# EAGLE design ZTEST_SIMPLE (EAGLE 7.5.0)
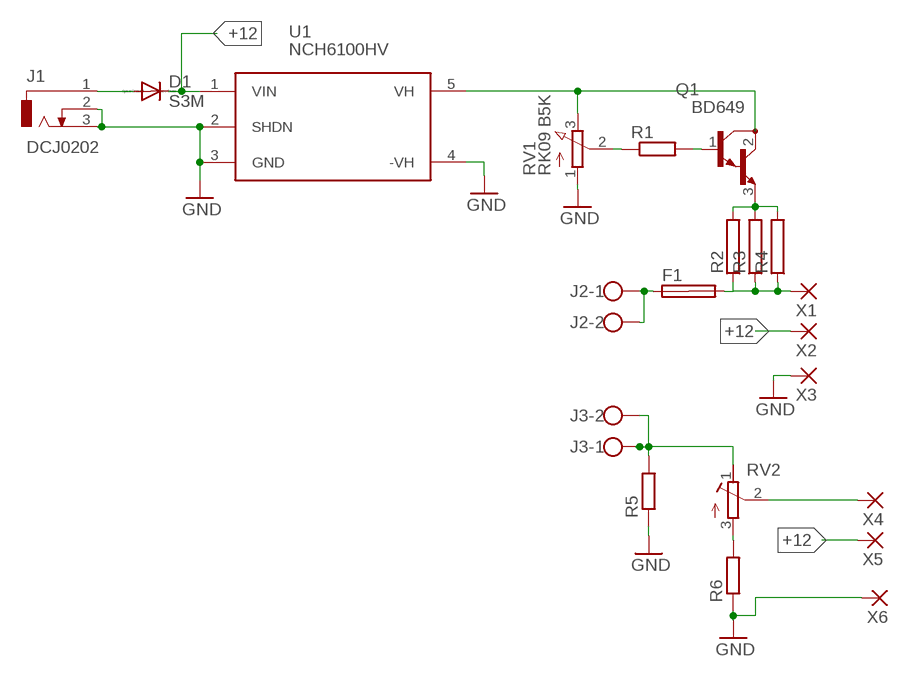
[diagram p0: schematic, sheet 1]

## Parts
D1  S3M  [SMC]
F1  SHK20L  [SHK20L]
J1  DCJ0202  [DCJ0202]
J2  W237-102  [W237-102]
J3  W237-102  [W237-102]
Q1  BD649  [TO220]
R1  R-EU_0207/10  [0207/10]
R2  RAC05  [AC05]
R3  RAC05  [AC05]
R4  RAC05  [AC05]
R5  R-EU_0411/12  [0411/12]
R6  R-EU_0207/10  [0207/10]
RV1  RK09 B5K  PV09A  [PTV09]
RV2  R-TRIMM-3386-F  [R-TRIMM-3386F]
U1  NCH6100HV  [NCH6100HV]
X1  2,54/1,1  [2,54/1,1]
X2  2,54/1,1  [2,54/1,1]
X3  2,54/1,1  [2,54/1,1]
X4  2,54/1,1  [2,54/1,1]
X5  2,54/1,1  [2,54/1,1]
X6  2,54/1,1  [2,54/1,1]

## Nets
+12: D1.C U1.1(VIN) X2.1(P) X5.1(P)
GND: J1.2 J1.3 R5.1 R6.1 RV1.1(A) U1.2(SHDN) U1.3(GND) U1.4(-VH) X3.1(P) X6.1(P)
N$2: D1.A J1.1
N$3: Q1.2(C) RV1.3(E) U1.5(VH)
N$4: Q1.1(B) R1.2
N$5: R1.1 RV1.2(S)
N$6: Q1.3(E) R2.2 R3.2 R4.2
N$7: F1.2A R2.1 R3.1 R4.1 X1.1(P)
N$8: F1.1A J2.1 J2.2
N$9: J3.1 J3.2 R5.2 RV2.1(A)
N$32: R6.2 RV2.3(E)
N$33: RV2.2(S) X4.1(P)
Unconnected: F1.1B F1.2B

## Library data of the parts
D1 = diode:S3M
F1 = fuse:SHK20L: FUSE HOLDER 5 x 20 mm, SH contact, SHH1 Schukat, E1073 Buerklin; OC_FARNELL: unknown; OC_NEWARK: unknown
J1 = con-jack:DCJ0202: DC POWER JACK Source: DCJ0202.pdf; OC_FARNELL: unknown; OC_NEWARK: unknown
J2 J3 = con-wago-500:W237-102: WAGO SCREW CLAMP; MPN: 237-102; OC_FARNELL: unknown; OC_NEWARK: 70K9898
Q1 = transistor:BD649: NPN BIPOLAR DARLINGTON TRANSISTOR
R1 R5 R6 = rcl:R-EU_: RESISTOR, European symbol
R2-R4 = resistor-power:R: Power Resitor; OC_FARNELL: unknown; OC_NEWARK: unknown
RV1 = pot:PV09A
RV2 = rcl:R-TRIMM-3386-F
U1 = dc-dc-converter:NCH6100HV
X1-X6 = wirepad:2,54/1,1: THROUGH-HOLE PAD

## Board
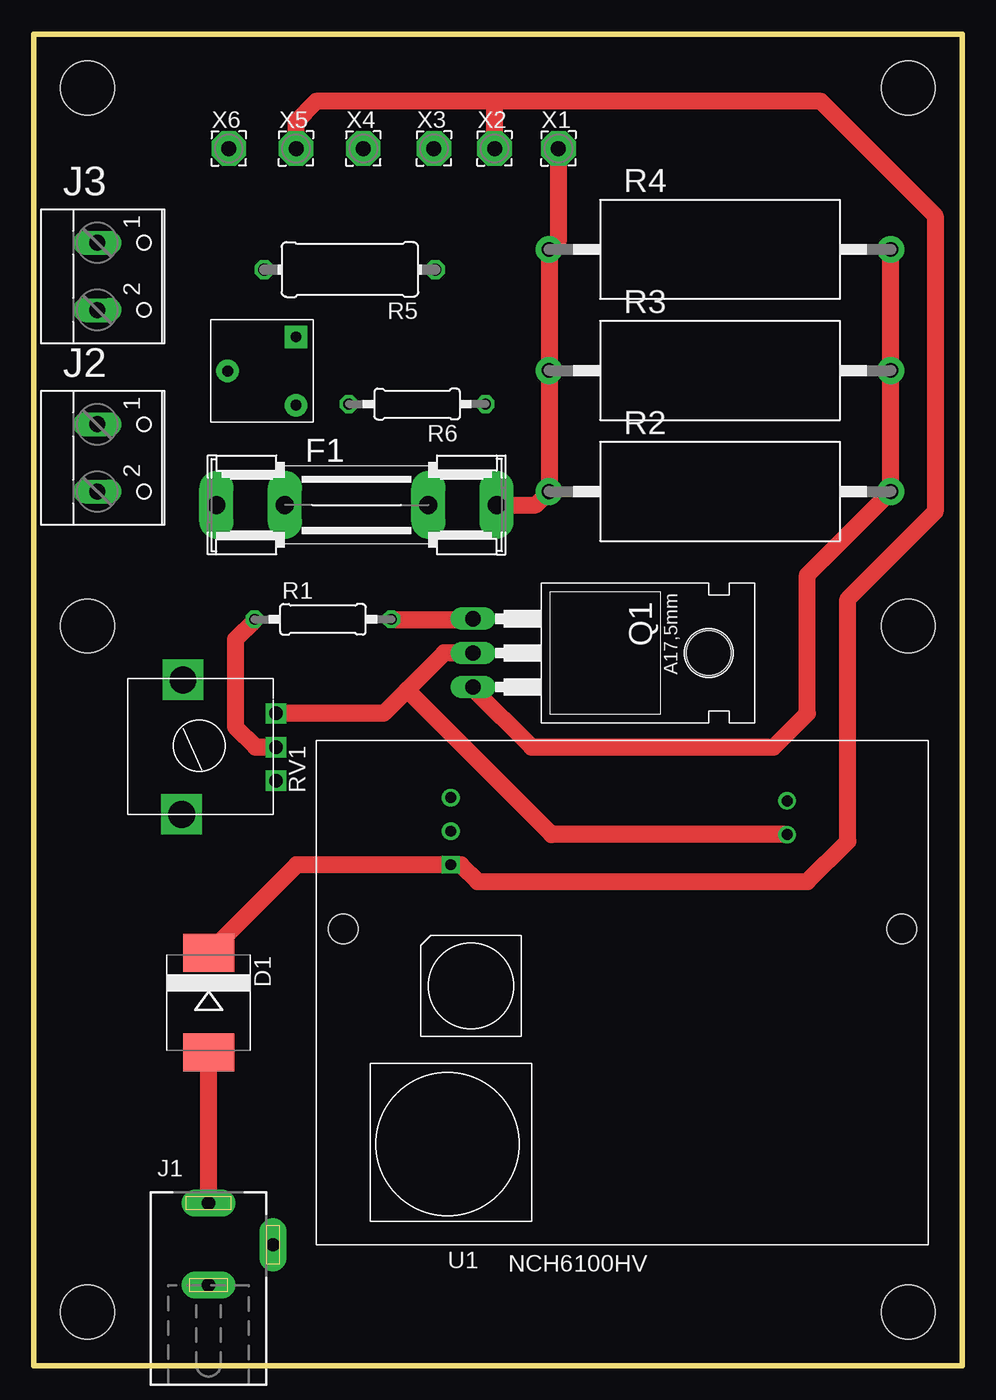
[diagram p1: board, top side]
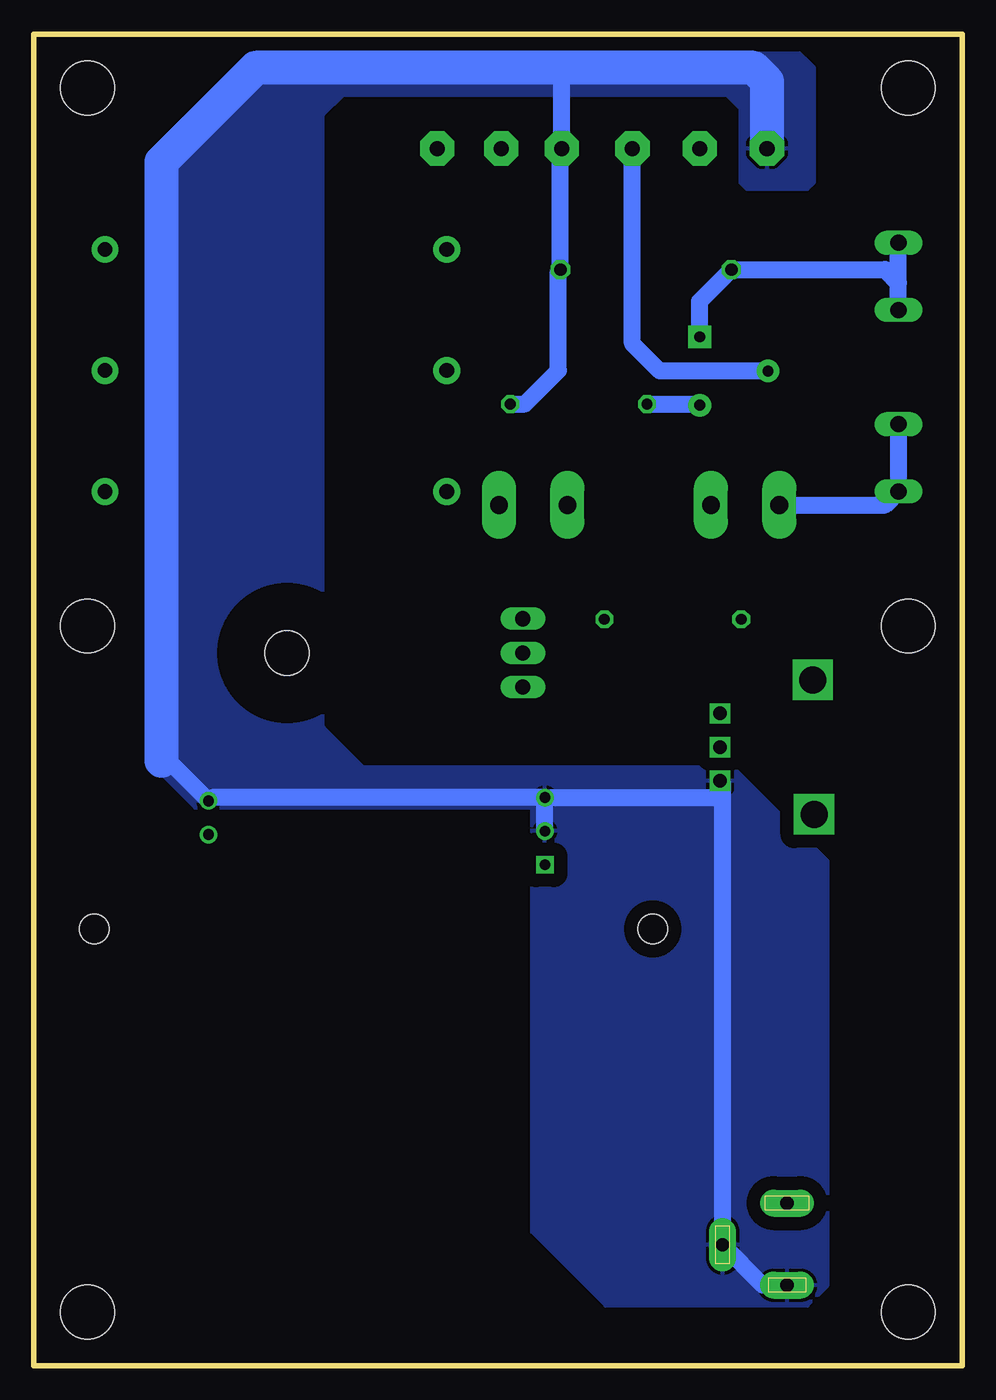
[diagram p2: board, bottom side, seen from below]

Size 69 x 99 mm. Coordinates in mm from the lower left corner, seen from the top.
Outline: 0,0 69,0 69,99 0,99 0,0
Copper layers (1*16): Top 0.035mm / dielectric 1.5mm / Bottom 0.035mm
Design rules "default": minimum track width 10mil, minimum drill 24mil, track to track 8mil, track to pad 8mil, pad to pad 8mil, via to via 8mil, smd to smd 8mil, copper to edge 40mil, drill to drill 8mil, minimum pad ring 10mil, minimum via ring 8mil, stop-mask expansion 4mil, vias tented up to drill 0mil, thermal gap 10mil
Holes 4 mm at 65,4 4,4 4,95 65,95 4,55 65,55

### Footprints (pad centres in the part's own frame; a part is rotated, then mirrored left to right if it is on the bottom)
SMC = smd 2.8 x 3.8: A 3.7,0; C -3.7,0
SHK20L = drill 1.321 pad 2.54 long: 1A -10.414,0; 1B -5.334,0; 2A 10.414,0; 2B 5.334,0
DCJ0202 = drill 1 pad 2 long: 1 0,3.1; 2 4.8,0; 3 0,-3
W237-102 = drill 1.194 long: 1 -2.5,-1.27; 2 2.5,-1.27
TO220 = drill 1.118 long: 1 -2.54,-6.35; 2 0,-6.35; 3 2.54,-6.35 | hole 3.302: 0,11.176
0207/10 = drill 0.813 octagon: 1 -5.08,0; 2 5.08,0
AC05 = drill 1.1 pad 2: 1 -12.7,0; 2 12.7,0
0411/12 = drill 0.914 octagon: 1 -6.35,0; 2 6.35,0
PTV09 = drill 1 square: 1 -2.5,0; 2 0,0; 3 2.5,0 | drill 2 square: P$4 -5,7; P$5 5,6.9
R-TRIMM-3386F = drill 0.8 pad 1.676 square: 1 0,0 | drill 0.8 pad 1.676: 2 5.08,2.54; 3 0,5.08
NCH6100HV = drill 0.8 square: 1 10,28.25 | drill 0.8: 2 10,30.75; 3 10,33.25; 4 35,33; 5 35,30.5 | hole 2.2: 2,23.5; 43.5,23.5
2,54/1,1 = drill 1.118 pad 2.54 octagon: 1 0,0

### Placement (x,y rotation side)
D1  13,27 270 top
F1  24,64 0 top
J1  13,9 0 top
J2  6,67.5 270 top
J3  6,81 270 top
Q1  39,53 270 top
R1  21.5,55.5 0 top
R2  51,65 0 top
R3  51,74 0 top
R4  51,83 0 top
R5  23.5,81.5 180 top
R6  28.5,71.5 180 top
RV1  18,46 90 top
RV2  19.5,76.5 180 top
U1  21,9 0 top
X1  39,90.5 0 top
X2  34.25,90.5 0 top
X3  29.75,90.5 0 top
X4  24.5,90.5 0 top
X5  19.5,90.5 0 top
X6  14.5,90.5 0 top

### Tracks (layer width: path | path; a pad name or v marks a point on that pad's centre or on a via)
+12
  Top 1.27: D1.C 19.55,37.25 U1.1 31.75,37.25 33,36 57.5,36 60.5,39 60.5,57 67,63.5 67,85.5 58.5,94 34,94 | X5.1 19.5,92.5 21,94 34,94 | X2.1 34.25,93.75 34,94
GND
  Bottom 1.27: J1.3 14.8,6 J1.2 17.8,42 | 17.8,42 17.8,43.3 RV1.1 | U1.2 U1.3 | U1.3 18.05,42.25 17.8,42 | U1.3 55.75,42.25 U1.4 59,45 59.5,45 | 30,96.5 29.75,96.25 X3.1 29.85,90.4 R5.1 30,81.35 30,74 32.5,71.5 R6.1
  Bottom 2.54: X6.1 14.5,95.5 15.5,96.5 30,96.5 52.5,96.5 59.5,89.5 59.5,45
  pour Bottom (isolate 1): 11,90 11,96.5 12.5,98 52.5,98 60.5,90 60.5,45 57,41.5 32,41.5 32,39 32,10 26.5,4.5 11.5,4.5 10,6 10,37.5 17,44.5 44.5,44.5 47.5,47.5 47.5,93 46,94.5 17.5,94.5 16.5,93.5 16.5,88 16,87.5 11.5,87.5 11,88
N$2
  Top 1.27: J1.1 D1.A
N$3
  Top 1.27: Q1.2 30.5,53 27.75,50.25 | 27.75,50.25 26,48.5 RV1.3 | U1.5 38.5,39.5 27.75,50.25
N$4
  Top 1.27: R1.2 32.61,55.5 Q1.1
N$5
  Top 1.27: R1.1 16.42,55.42 15,54 15,47.5 16.5,46 RV1.2
N$6
  Top 1.27: Q1.3 32.65,50.35 37,46 55,46 57.5,48.5 57.5,58.8 R2.2 R3.2 R4.2
N$7
  Top 1.27: X1.1 39,83.7 R4.1 R3.1 R2.1 37.3,64 F1.2A
N$8
  Bottom 1.27: F1.1A 5.73,64 J2.2 J2.1
N$9
  Bottom 1.27: J3.2 4.73,80.5 | 4.73,80.5 J3.1 | 4.73,80.5 5.73,81.5 R5.2 19.5,79.15 RV2.1
N$32
  Bottom 1.27: R6.2 19.58,71.5 RV2.3
N$33
  Bottom 1.27: RV2.2 22.46,73.96 24.5,76 X4.1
